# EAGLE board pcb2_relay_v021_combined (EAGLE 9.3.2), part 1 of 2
2022-05-20: PCB made by JLCPCB
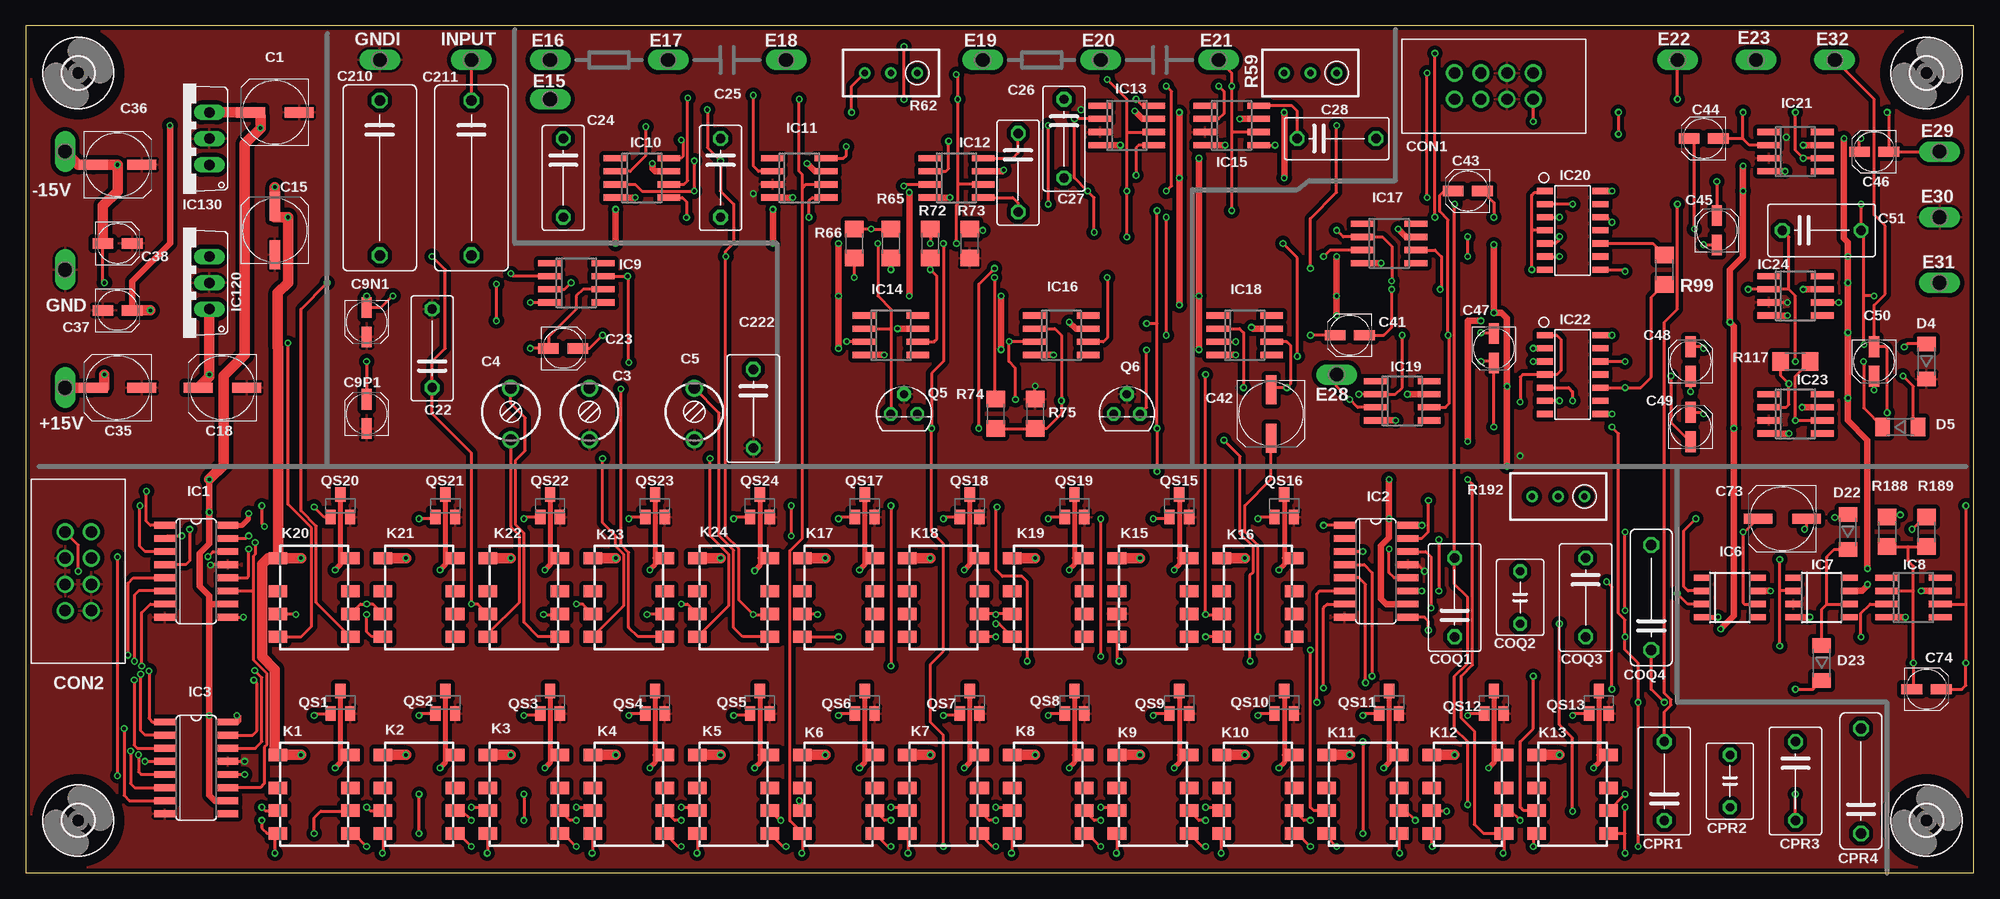
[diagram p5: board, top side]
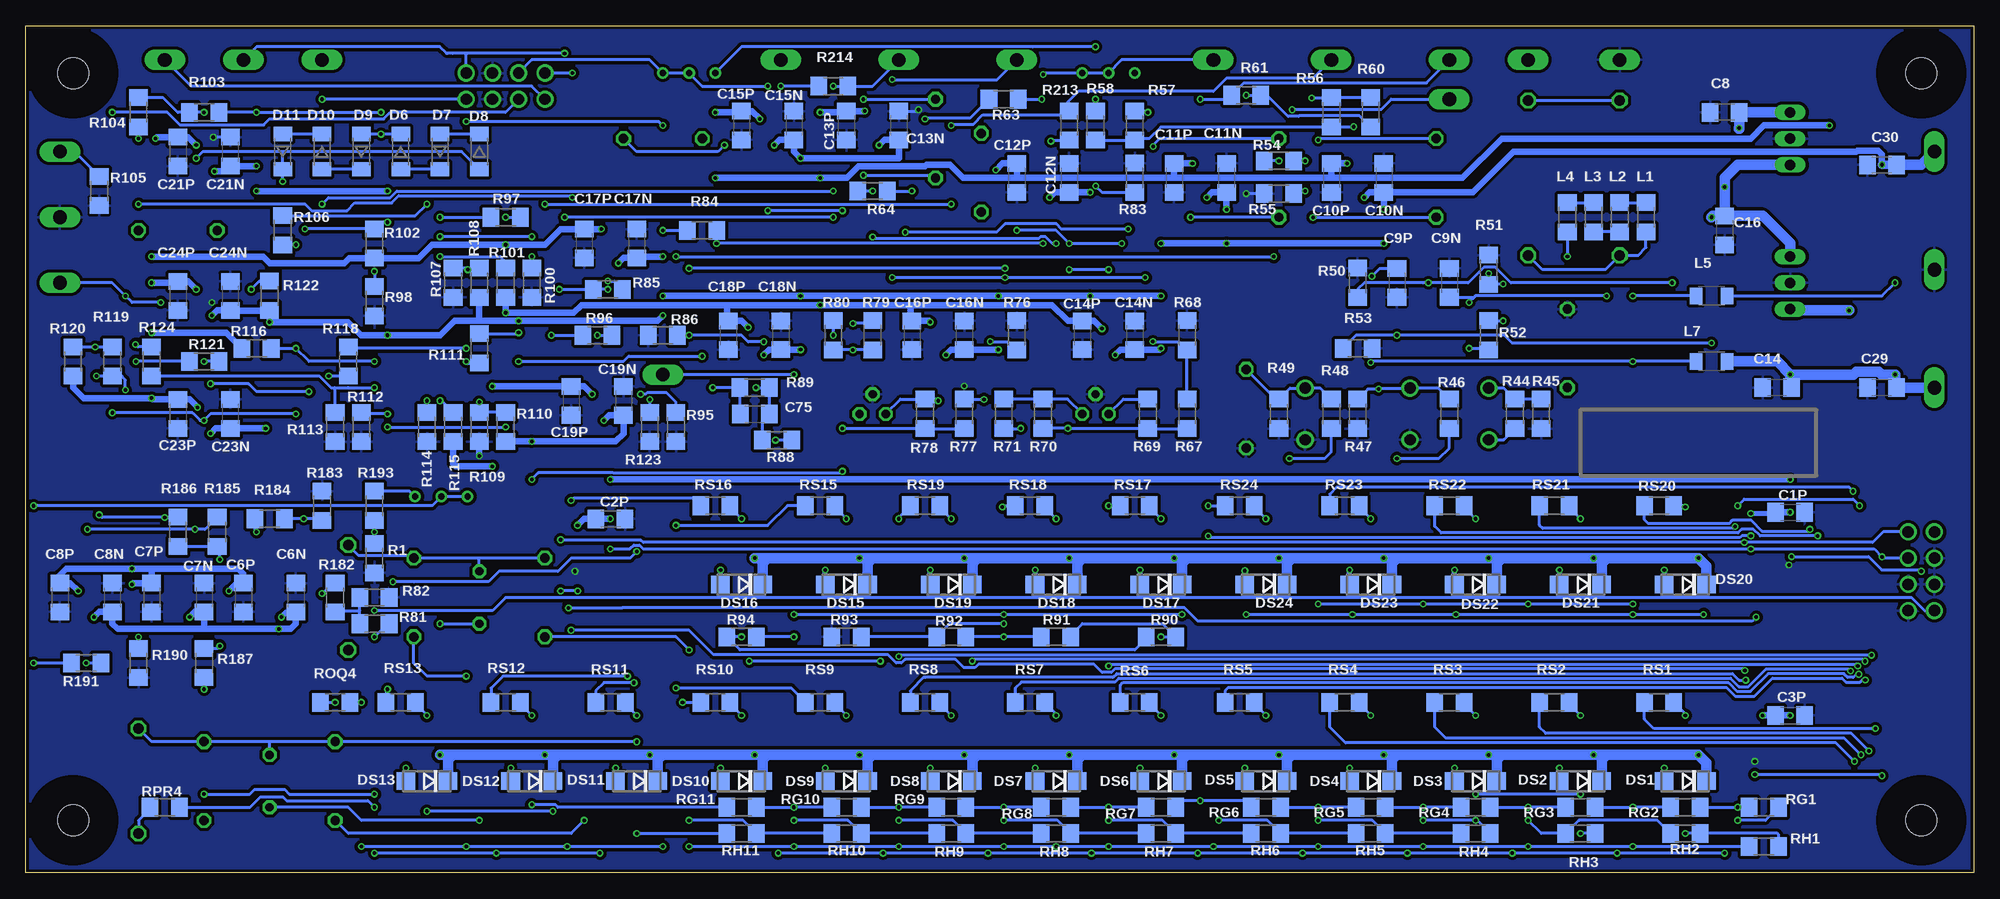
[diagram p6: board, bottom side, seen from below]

Size 188.72 x 82.04 mm. Coordinates in mm from the lower left corner, seen from the top.
Outline: 0,0 188.72,0 188.72,82.04 0,82.04 0,0
Copper layers (1*16): Top 0.035mm / dielectric 1.5mm / Bottom 0.035mm
Design rules "ITEADstudio_DRC for Eagle v6": minimum track width 6mil, minimum drill 12mil, track to track 6mil, track to pad 6mil, pad to pad 6mil, via to via 6mil, smd to smd 0mil, copper to edge 10mil, drill to drill 10mil, minimum pad ring 10mil, minimum via ring 6mil, stop-mask expansion 2mil, vias tented up to drill 100mil, thermal gap 10mil

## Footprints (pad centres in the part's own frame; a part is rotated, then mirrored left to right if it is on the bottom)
P1-13Y = drill 1.321 pad 1.905 long: TP 0,0
UD-6,3X5,8_NICHICON = smd 2.8 x 1: + 2.35,0; - -2.35,0
C1206 = smd 1.6 x 1.8: 1 -1.4,0; 2 1.4,0
CTRIM3050.504 = drill 1.1: 1 -2.5,0; 2 2.5,0
UD-4X5,8_NICHICON = smd 2 x 1: + 1.425,0; - -1.425,0
C075-042X103 = drill 0.914 octagon: 1 -3.81,0; 2 3.81,0
C075-052X106 = drill 0.914 octagon: 1 -3.81,0; 2 3.81,0
C150-072X183 = drill 1.016 octagon: 1 -7.493,0; 2 7.493,0
61200821621 = drill 1.1: 1 -2.54,-1.27; 2 -2.54,1.27; 3 0,-1.27; 4 0,1.27; 5 2.54,-1.27; 6 2.54,1.27; 7 5.08,-1.27; 8 5.08,1.27
C050-045X075 = drill 0.813 octagon: 1 -2.54,0; 2 2.54,0
C102-043X133 = drill 1.016 octagon: 1 -5.08,0; 2 5.08,0
SOD80 = smd 1.4 x 1.8: 1 -1.7,0; 2 1.7,0
DO214AC = smd 1.8 x 1.7: A 2.05,0; C -2.05,0
SO16 = smd 0.66 x 2.032: 1 -4.445,-3.073; 2 -3.175,-3.073; 3 -1.905,-3.073; 4 -0.635,-3.073; 5 0.635,-3.073; 6 1.905,-3.073; 7 3.175,-3.073; 8 4.445,-3.073; 9 4.445,3.073; 10 3.175,3.073; 11 1.905,3.073; 12 0.635,3.073; 13 -0.635,3.073; 14 -1.905,3.073; 15 -3.175,3.073; 16 -4.445,3.073
SOIC8 = smd 0.6 x 1.5: 1 -1.905,-2.75; 2 -0.635,-2.75; 3 0.635,-2.75; 4 1.905,-2.75; 5 1.905,2.75; 6 0.635,2.75; 7 -0.635,2.75; 8 -1.905,2.75
SO08 = smd 0.6 x 2.2: 1 -1.905,-2.6; 2 -0.635,-2.6; 3 0.635,-2.6; 4 1.905,-2.6; 5 1.905,2.6; 6 0.635,2.6; 7 -0.635,2.6; 8 -1.905,2.6
SOIC-14 = smd 0.6 x 1.55: 1 -3.81,-2.7; 2 -2.54,-2.7; 3 -1.27,-2.7; 4 0,-2.7; 5 1.27,-2.7; 6 2.54,-2.7; 7 3.81,-2.7; 8 3.81,2.7; 9 2.54,2.7; 10 1.27,2.7; 11 0,2.7; 12 -1.27,2.7; 13 -2.54,2.7; 14 -3.81,2.7
TO220V = drill 1.016 long: 1 -2.54,-2.54; 2 0,-2.54; 3 2.54,-2.54
G6K-2F-Y = smd 1.2 x 1.8: 1 -3.8,-3.5; 2 -0.6,-3.5; 3 1.6,-3.5; 4 3.8,-3.5; 5 3.8,3.5; 6 1.6,3.5; 7 -0.6,3.5; 8 -3.8,3.5
FB1206 = smd 1.6 x 1.803: 1 -1.422,0; 2 1.422,0
L3216C = smd 1.2 x 1.6: 1 -1.5,0; 2 1.5,0
TO92G = drill 0.813 octagon: D -1.27,0; G 1.27,0; S 0,1.905
SOT23 = smd 1 x 1.4: 1 -0.95,-1.1; 2 0.95,-1.1; 3 0,1.1
R1206 = smd 1.6 x 1.803: 1 -1.422,0; 2 1.422,0
RTRIM3296W = drill 0.61: 1 0,-2.54; 2 0,0; 3 0,2.54
3,0 = hole 3: 0,0

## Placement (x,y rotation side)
+15V  TPPAD1-13Y  [P1-13Y]  3.81,46.99 0 top
-15V  TPPAD1-13Y  [P1-13Y]  3.81,69.85 0 top
C1  100u/16V  [UD-6,3X5,8_NICHICON]  24.13,73.66 180 top
C1P  100n  [C1206]  17.78,34.92 0 bottom
C2P  100n  [C1206]  132.08,34.29 0 bottom
C3  30p  [CTRIM3050.504]  54.61,44.45 90 top
C3P  100n  [C1206]  17.78,15.24 0 bottom
C4  5p  [CTRIM3050.504]  46.99,44.45 90 top
C5  30p  [CTRIM3050.504]  64.77,44.45 90 top
C6N  100n  [C1206]  162.56,26.67 270 bottom
C6P  100n  [C1206]  167.64,26.67 270 bottom
C7N  100n  [C1206]  171.45,26.67 270 bottom
C7P  100n  [C1206]  176.53,26.67 270 bottom
C8  100n  [C1206]  24.13,73.66 180 bottom
C8N  100n  [C1206]  180.34,26.67 270 bottom
C8P  100n  [C1206]  185.42,26.67 270 bottom
C9N  100n  [C1206]  50.8,57.15 270 bottom
C9N1  10u/25V  [UD-4X5,8_NICHICON]  33.02,53.34 270 top
C9P  100n  [C1206]  55.88,57.15 270 bottom
C9P1  10u/25V  [UD-4X5,8_NICHICON]  33.02,44.45 90 top
C10N  100n  [C1206]  57.15,67.31 270 bottom
C10P  100n  [C1206]  62.23,67.31 270 bottom
C11N  100n  [C1206]  72.39,67.31 270 bottom
C11P  100n  [C1206]  77.47,67.31 270 bottom
C12N  100n  [C1206]  87.63,67.31 270 bottom
C12P  100n  [C1206]  92.71,67.31 270 bottom
C13N  100n  [C1206]  104.14,72.39 270 bottom
C13P  100n  [C1206]  109.22,72.39 270 bottom
C14  100n  [C1206]  19.05,46.99 180 bottom
C14N  100n  [C1206]  81.28,52.07 270 bottom
C14P  100n  [C1206]  86.36,52.07 270 bottom
C15  100u/16V  [UD-6,3X5,8_NICHICON]  24.13,62.23 90 top
C15N  100n  [C1206]  114.3,72.39 270 bottom
C15P  100n  [C1206]  119.38,72.39 270 bottom
C16  100n  [C1206]  24.13,62.23 270 bottom
C16N  100n  [C1206]  97.79,52.07 270 bottom
C16P  100n  [C1206]  102.87,52.07 270 bottom
C17N  100n  [C1206]  129.54,60.96 270 bottom
C17P  100n  [C1206]  134.62,60.96 270 bottom
C18  100u/16V  [UD-6,3X5,8_NICHICON]  19.05,46.99 180 top
C18N  100n  [C1206]  115.57,52.07 270 bottom
C18P  100n  [C1206]  120.65,52.07 270 bottom
C19N  100n  [C1206]  130.81,45.72 270 bottom
C19P  100n  [C1206]  135.89,45.72 270 bottom
C21N  100n  [C1206]  168.91,69.85 270 bottom
C21P  100n  [C1206]  173.99,69.85 270 bottom
C22  47p  [C075-042X103]  39.37,50.8 90 top
C23  10u/25V  [UD-4X5,8_NICHICON]  52.07,50.8 0 top
C23N  100n  [C1206]  168.91,44.45 270 bottom
C23P  100n  [C1206]  173.99,44.45 270 bottom
C24  10p  [C075-042X103]  52.07,67.31 270 top
C24N  100n  [C1206]  168.91,55.88 270 bottom
C24P  100n  [C1206]  173.99,55.88 270 bottom
C25  15p  [C075-042X103]  67.31,67.31 270 top
C26  22p  [C075-042X103]  96.14,67.82 270 top
C27  15p  [C075-042X103]  100.58,71.12 270 top
C28  22p  [C075-042X103]  127,71.12 0 top
C29  100n  [C1206]  8.89,46.99 180 bottom
C30  100n  [C1206]  8.89,68.58 0 bottom
C35  100u/16V  [UD-6,3X5,8_NICHICON]  8.89,46.99 180 top
C36  100u/16V  [UD-6,3X5,8_NICHICON]  8.89,68.58 0 top
C37  1u/50V  [UD-4X5,8_NICHICON]  8.89,54.48 0 top
C38  1u/50V  [UD-4X5,8_NICHICON]  8.89,60.96 0 top
C41  10u/25V  [UD-4X5,8_NICHICON]  128.27,52.07 180 top
C42  100u/16V  [UD-6,3X5,8_NICHICON]  120.65,44.45 270 top
C43  10u/25V  [UD-4X5,8_NICHICON]  139.7,66.04 180 top
C44  1u/50V  [UD-4X5,8_NICHICON]  162.56,71.12 180 top
C45  10u/25V  [UD-4X5,8_NICHICON]  163.83,62.23 90 top
C46  10u/25V  [UD-4X5,8_NICHICON]  179.07,69.85 180 top
C47  10u/25V  [UD-4X5,8_NICHICON]  142.24,50.8 270 top
C48  1u/50V  [UD-4X5,8_NICHICON]  161.29,49.53 90 top
C49  10u/25V  [UD-4X5,8_NICHICON]  161.29,43.18 90 top
C50  1u/50V  [UD-4X5,8_NICHICON]  179.07,49.53 270 top
C51  220n  [C075-052X106]  173.99,62.23 0 top
C73  100u/16V  [UD-6,3X5,8_NICHICON]  170.18,34.29 180 top
C74  1u/50V  [UD-4X5,8_NICHICON]  184.15,17.78 0 top
C75  2p  [C1206]  118.11,44.45 0 bottom
C210  1u  [C150-072X183]  34.29,67.31 270 top
C211  1u  [C150-072X183]  43.18,67.31 270 top
C222  68p  [C075-052X106]  70.48,44.96 270 top
CON1  PCB2_IO  [61200821621]  140.97,76.2 0 top
CON2  UC_IO  [61200821621]  5.08,27.94 90 top
COQ1  220n  [C075-052X106]  138.43,26.67 90 top
COQ2  22n  [C050-045X075]  144.78,26.67 90 top
COQ3  2n2  [C075-052X106]  151.13,26.67 270 top
COQ4  200p  [C102-043X133]  157.48,26.67 90 top
CPR1  220n  [C075-052X106]  158.75,8.89 90 top
CPR2  22n  [C050-045X075]  165.1,8.89 90 top
CPR3  2n2  [C075-052X106]  171.45,8.89 270 top
CPR4  200p  [C102-043X133]  177.8,8.89 90 top
D4  1N4148  [SOD80]  184.15,49.53 90 top
D5  1N4148  [SOD80]  181.61,43.18 0 top
D6  1N4148  [SOD80]  152.4,69.85 270 bottom
D7  1N4148  [SOD80]  148.59,69.85 90 bottom
D8  1N4148  [SOD80]  144.78,69.85 270 bottom
D9  1N4148  [SOD80]  156.21,69.85 90 bottom
D10  1N4148  [SOD80]  160.02,69.85 270 bottom
D11  1N4148  [SOD80]  163.83,69.85 90 bottom
D22  1N4148  [SOD80]  176.53,33.02 90 top
D23  1N4148  [SOD80]  173.99,20.32 90 top
DS1  M7  [DO214AC]  27.94,8.89 180 bottom
DS2  M7  [DO214AC]  38.1,8.89 180 bottom
DS3  M7  [DO214AC]  48.26,8.89 180 bottom
DS4  M7  [DO214AC]  58.42,8.89 180 bottom
DS5  M7  [DO214AC]  68.58,8.89 180 bottom
DS6  M7  [DO214AC]  78.74,8.89 180 bottom
DS7  M7  [DO214AC]  88.9,8.89 180 bottom
DS8  M7  [DO214AC]  99.06,8.89 180 bottom
DS9  M7  [DO214AC]  109.22,8.89 180 bottom
DS10  M7  [DO214AC]  119.38,8.89 180 bottom
DS11  M7  [DO214AC]  129.54,8.89 180 bottom
DS12  M7  [DO214AC]  139.7,8.89 180 bottom
DS13  M7  [DO214AC]  149.86,8.89 180 bottom
DS15  M7  [DO214AC]  109.22,27.94 180 bottom
DS16  M7  [DO214AC]  119.38,27.94 180 bottom
DS17  M7  [DO214AC]  78.74,27.94 180 bottom
DS18  M7  [DO214AC]  88.9,27.94 180 bottom
DS19  M7  [DO214AC]  99.06,27.94 180 bottom
DS20  M7  [DO214AC]  27.94,27.94 180 bottom
DS21  M7  [DO214AC]  38.1,27.94 180 bottom
DS22  M7  [DO214AC]  48.26,27.94 180 bottom
DS23  M7  [DO214AC]  58.42,27.94 180 bottom
DS24  M7  [DO214AC]  68.58,27.94 180 bottom
E15  TPPAD1-13Y  [P1-13Y]  50.8,74.93 90 top
E16  TPPAD1-13Y  [P1-13Y]  50.8,78.74 90 top
E17  TPPAD1-13Y  [P1-13Y]  62.23,78.74 90 top
E18  TPPAD1-13Y  [P1-13Y]  73.66,78.74 90 top
E19  TPPAD1-13Y  [P1-13Y]  92.71,78.74 90 top
E20  TPPAD1-13Y  [P1-13Y]  104.14,78.74 270 top
E21  TPPAD1-13Y  [P1-13Y]  115.57,78.74 270 top
E22  TPPAD1-13Y  [P1-13Y]  160.02,78.74 90 top
E23  TPPAD1-13Y  [P1-13Y]  167.64,78.74 90 top
E28  TPPAD1-13Y  [P1-13Y]  127,48.26 270 top
E29  TPPAD1-13Y  [P1-13Y]  185.42,69.85 90 top
E30  TPPAD1-13Y  [P1-13Y]  185.42,63.5 90 top
E31  TPPAD1-13Y  [P1-13Y]  185.42,57.15 90 top
E32  TPPAD1-13Y  [P1-13Y]  175.26,78.74 90 top
GND  TPPAD1-13Y  [P1-13Y]  3.81,58.42 0 top
GNDI  TPPAD1-13Y  [P1-13Y]  34.29,78.74 90 top
IC1  74HC595D  [SO16]  16.51,29.21 270 top
IC2  74HC595D  [SO16]  130.81,29.21 270 top
IC3  74HC595D  [SO16]  16.51,10.16 270 top
IC6  LM318D  [SOIC8]  165.1,26.67 270 top
IC7  LM318D  [SOIC8]  173.99,26.67 270 top
IC8  LM741D  [SO08]  182.88,26.67 270 top
IC9  NE5534AD  [SO08]  53.34,57.15 270 top
IC10  NE5534AD  [SO08]  59.69,67.31 270 top
IC11  NE5534AD  [SO08]  74.93,67.31 270 top
IC12  NE5534AD  [SO08]  90.17,67.31 270 top
IC13  NE5534AD  [SO08]  106.68,72.39 270 top
IC14  NE5534AD  [SO08]  83.82,52.07 270 top
IC15  NE5534AD  [SO08]  116.84,72.39 270 top
IC16  NE5534AD  [SO08]  100.33,52.07 270 top
IC17  NE5534AD  [SO08]  132.08,60.96 270 top
IC18  LM318D  [SO08]  118.11,52.07 270 top
IC19  LM318D  [SO08]  133.35,45.72 270 top
IC20  MC1496D  [SOIC-14]  149.86,62.23 270 top
IC21  LM318D  [SO08]  171.45,69.85 270 top
IC22  MC1496D  [SOIC-14]  149.86,48.26 270 top
IC23  LM318D  [SO08]  171.45,44.45 270 top
IC24  LF356D  [SO08]  171.45,55.88 270 top
IC120  7812TV  [TO220V]  15.24,57.15 90 top
IC130  7805TV  [TO220V]  15.24,71.12 90 top
INPUT  TPPAD1-13Y  [P1-13Y]  43.18,78.74 90 top
K1  G6K-2F-Y  [G6K-2F-Y]  27.94,7.62 270 top
K2  G6K-2F-Y  [G6K-2F-Y]  38.1,7.62 270 top
K3  G6K-2F-Y  [G6K-2F-Y]  48.26,7.62 270 top
K4  G6K-2F-Y  [G6K-2F-Y]  58.42,7.62 270 top
K5  G6K-2F-Y  [G6K-2F-Y]  68.58,7.62 270 top
K6  G6K-2F-Y  [G6K-2F-Y]  78.74,7.62 270 top
K7  G6K-2F-Y  [G6K-2F-Y]  88.9,7.62 270 top
K8  G6K-2F-Y  [G6K-2F-Y]  99.06,7.62 270 top
K9  G6K-2F-Y  [G6K-2F-Y]  109.22,7.62 270 top
K10  G6K-2F-Y  [G6K-2F-Y]  119.38,7.62 270 top
K11  G6K-2F-Y  [G6K-2F-Y]  129.54,7.62 270 top
K12  G6K-2F-Y  [G6K-2F-Y]  139.7,7.62 270 top
K13  G6K-2F-Y  [G6K-2F-Y]  149.86,7.62 270 top
K15  G6K-2F-Y  [G6K-2F-Y]  109.22,26.67 270 top
K16  G6K-2F-Y  [G6K-2F-Y]  119.38,26.67 270 top
K17  G6K-2F-Y  [G6K-2F-Y]  78.74,26.67 270 top
K18  G6K-2F-Y  [G6K-2F-Y]  88.9,26.67 270 top
K19  G6K-2F-Y  [G6K-2F-Y]  99.06,26.67 270 top
K20  G6K-2F-Y  [G6K-2F-Y]  27.94,26.67 270 top
K21  G6K-2F-Y  [G6K-2F-Y]  38.1,26.67 270 top
K22  G6K-2F-Y  [G6K-2F-Y]  48.26,26.67 270 top
K23  G6K-2F-Y  [G6K-2F-Y]  58.42,26.67 270 top
K24  G6K-2F-Y  [G6K-2F-Y]  68.58,26.67 270 top
L1  600  [FB1206]  31.75,63.5 270 bottom
L2  600  [FB1206]  34.29,63.5 270 bottom
L3  600  [FB1206]  36.83,63.5 270 bottom
L4  600  [FB1206]  39.37,63.5 270 bottom
L5  10u  [L3216C]  25.4,55.88 180 bottom
L7  10u  [L3216C]  25.4,49.53 180 bottom
Q5  2N4091  [TO92G]  85.09,44.45 0 top
Q6  2N4091  [TO92G]  106.68,44.45 0 top
QS1  SS8050  [SOT23]  30.48,16.51 0 top
QS2  SS8050  [SOT23]  40.64,16.51 0 top
QS3  SS8050  [SOT23]  50.8,16.51 0 top
QS4  SS8050  [SOT23]  60.96,16.51 0 top
QS5  SS8050  [SOT23]  71.12,16.51 0 top
QS6  SS8050  [SOT23]  81.28,16.51 0 top
QS7  SS8050  [SOT23]  91.44,16.51 0 top
QS8  SS8050  [SOT23]  101.6,16.51 0 top
QS9  SS8050  [SOT23]  111.76,16.51 0 top
QS10  SS8050  [SOT23]  121.92,16.51 0 top
QS11  SS8050  [SOT23]  132.08,16.51 0 top
QS12  SS8050  [SOT23]  142.24,16.51 0 top
QS13  SS8050  [SOT23]  152.4,16.51 0 top
QS15  SS8050  [SOT23]  111.76,35.56 0 top
QS16  SS8050  [SOT23]  121.92,35.56 0 top
QS17  SS8050  [SOT23]  81.28,35.56 0 top
QS18  SS8050  [SOT23]  91.44,35.56 0 top
QS19  SS8050  [SOT23]  101.6,35.56 0 top
QS20  SS8050  [SOT23]  30.48,35.56 0 top
QS21  SS8050  [SOT23]  40.64,35.56 0 top
QS22  SS8050  [SOT23]  50.8,35.56 0 top
QS23  SS8050  [SOT23]  60.96,35.56 0 top
QS24  SS8050  [SOT23]  71.12,35.56 0 top
R1  3K3  [R1206]  154.94,30.48 90 bottom
R44  68K1  [R1206]  44.45,44.45 90 bottom
R45  42K2  [R1206]  41.91,44.45 90 bottom
R46  90K9  [R1206]  50.8,44.45 90 bottom
R47  11K  [R1206]  59.69,44.45 90 bottom
R48  100K  [R1206]  62.23,44.45 90 bottom
R49  3K16  [R1206]  67.31,44.45 90 bottom
R50  100K  [R1206]  59.69,57.15 270 bottom
R51  1K  [R1206]  46.99,58.42 270 bottom
R52  2K05  [R1206]  46.99,52.07 270 bottom
R53  1M  [R1206]  59.69,50.8 180 bottom
R54  82K  [R1206]  67.31,68.96 180 bottom
R55  18K  [R1206]  67.31,65.79 0 bottom
R56  10K  [R1206]  62.23,73.66 90 bottom
R57  22k  [R1206]  81.28,72.39 90 bottom
R58  6K8  [R1206]  85.09,72.39 90 bottom
R59  5K  [RTRIM3296W]  124.46,77.47 90 top
R60  10K  [R1206]  58.42,73.66 270 bottom
R61  10K  [R1206]  70.48,75.31 180 bottom
R62  5K  [RTRIM3296W]  83.82,77.47 90 top
R63  10K  [R1206]  93.98,74.93 0 bottom
R64  10K  [R1206]  106.68,66.04 180 bottom
R65  82K  [R1206]  83.82,60.96 270 top
R66  150K  [R1206]  80.26,60.96 90 top
R67  10K  [R1206]  76.2,44.45 270 bottom
R68  270  [R1206]  76.2,52.07 270 bottom
R69  1K5  [R1206]  80.01,44.45 270 bottom
R70  750K  [R1206]  90.17,44.45 270 bottom
R71  10K  [R1206]  93.98,44.45 90 bottom
R72  560  [R1206]  87.63,60.96 270 top
R73  330  [R1206]  91.44,60.96 90 top
R74  560  [R1206]  93.98,44.45 90 top
R75  330  [R1206]  97.79,44.45 270 top
R76  270  [R1206]  92.71,52.07 270 bottom
R77  10K  [R1206]  97.79,44.45 270 bottom
R78  1K5  [R1206]  101.6,44.45 270 bottom
R79  750K  [R1206]  106.68,52.07 90 bottom
R80  10K  [R1206]  110.49,52.07 270 bottom
R81  27K  [R1206]  154.94,24.13 180 bottom
R82  4K7  [R1206]  154.94,26.67 0 bottom
R83  100  [R1206]  81.28,67.31 270 bottom
R84  2K2  [R1206]  123.19,62.23 0 bottom
R85  18K  [R1206]  132.33,56.52 0 bottom
R86  100K  [R1206]  127,52.07 0 bottom
R88  1K1  [R1206]  115.95,41.91 0 bottom
R89  10K  [R1206]  118.11,46.99 0 bottom
R90  7K5  [R1206]  78.74,22.86 0 bottom
R91  2K15  [R1206]  88.9,22.86 180 bottom
R92  750  [R1206]  99.06,22.86 180 bottom
R93  316  [R1206]  109.22,22.86 180 bottom
R94  6K2  [R1206]  119.38,22.86 180 bottom
R95  1K1  [R1206]  125.73,43.18 270 bottom
R96  10K  [R1206]  133.35,52.07 0 bottom
R97  15K  [R1206]  142.24,63.5 0 bottom
R98  100  [R1206]  154.94,55.37 270 bottom
R99  100  [R1206]  158.75,58.42 270 top
R100  15K  [R1206]  139.7,57.15 270 bottom
R101  100  [R1206]  142.24,57.15 90 bottom
R102  6K8  [R1206]  154.94,60.96 270 bottom
R103  1M  [R1206]  171.45,73.66 180 bottom
R104  470  [R1206]  177.8,73.66 270 bottom
R105  100K  [R1206]  181.61,66.04 270 bottom
R106  15K  [R1206]  163.83,62.23 270 bottom
R107  4K7  [R1206]  147.32,57.15 90 bottom
R108  4K7  [R1206]  144.78,57.15 270 bottom
R109  4K7  [R1206]  144.78,43.18 90 bottom
R110  4K7  [R1206]  142.24,43.18 270 bottom
R111  15K  [R1206]  144.78,50.8 90 bottom
R112  100  [R1206]  156.21,43.18 270 bottom
R113  100  [R1206]  158.75,43.18 270 bottom
R114  15K  [R1206]  149.86,43.18 270 bottom
R115  100  [R1206]  147.32,43.18 90 bottom
R116  6K8  [R1206]  166.37,50.8 180 bottom
R117  1M  [R1206]  171.45,49.53 0 top
R118  15K  [R1206]  157.48,49.53 270 bottom
R119  100K  [R1206]  180.34,49.53 270 bottom
R120  100K  [R1206]  184.15,49.53 90 bottom
R121  1M  [R1206]  171.45,49.53 0 bottom
R122  22M  [R1206]  165.1,55.88 90 bottom
R123  100K  [R1206]  128.27,43.18 90 bottom
R124  11K  [R1206]  176.53,49.53 90 bottom
R182  100  [R1206]  158.75,26.67 270 bottom
R183  1K  [R1206]  160.02,35.56 90 bottom
R184  1K  [R1206]  165.1,34.29 0 bottom
R185  1K  [R1206]  170.18,33.02 90 bottom
R186  1K  [R1206]  173.99,33.02 90 bottom
R187  1K  [R1206]  171.45,20.32 90 bottom
R188  10K  [R1206]  180.34,33.02 270 top
R189  20K  [R1206]  184.15,33.02 90 top
R190  6K8  [R1206]  177.8,20.32 90 bottom
R191  270K  [R1206]  182.88,20.32 180 bottom
R192  5K  [RTRIM3296W]  148.46,36.45 90 top
R193  4K7  [R1206]  154.94,35.56 90 bottom
R213  220  [R1206]  87.63,72.39 270 bottom
R214  220  [R1206]  110.49,76.2 180 bottom
RG1  7K5  [R1206]  20.32,6.35 180 bottom
RG2  5K62  [R1206]  27.94,6.35 180 bottom
RG3  6K19  [R1206]  38.1,6.35 180 bottom
RG4  3K83  [R1206]  48.26,6.35 180 bottom
RG5  3K48  [R1206]  58.42,6.35 180 bottom
RG6  2K15  [R1206]  68.58,6.35 180 bottom
RG7  1K96  [R1206]  78.74,6.35 180 bottom
RG8  1K78  [R1206]  88.9,6.35 180 bottom
RG9  1K1  [R1206]  99.06,6.35 180 bottom
RG10  1K  [R1206]  109.22,6.35 180 bottom
RG11  3K83  [R1206]  119.38,6.35 180 bottom
RH1  7K5  [R1206]  20.32,2.54 0 bottom
RH2  5K62  [R1206]  27.94,3.81 180 bottom
RH3  6K19  [R1206]  38.1,3.81 0 bottom
RH4  3K83  [R1206]  48.26,3.81 180 bottom
RH5  3K48  [R1206]  58.42,3.81 180 bottom
RH6  2K15  [R1206]  68.58,3.81 180 bottom
RH7  1K96  [R1206]  78.74,3.81 180 bottom
RH8  1K78  [R1206]  88.9,3.81 180 bottom
RH9  1K1  [R1206]  99.06,3.81 180 bottom
RH10  1K  [R1206]  109.22,3.81 180 bottom
RH11  3K83  [R1206]  119.38,3.81 180 bottom
ROQ4  180  [R1206]  158.75,16.51 180 bottom
RPR4  180  [R1206]  175.26,6.35 180 bottom
RS1  4K7  [R1206]  30.48,16.51 180 bottom
RS2  4K7  [R1206]  40.64,16.51 180 bottom
RS3  4K7  [R1206]  50.8,16.51 180 bottom
RS4  4K7  [R1206]  60.96,16.51 180 bottom
RS5  4K7  [R1206]  71.12,16.51 180 bottom
RS6  4K7  [R1206]  81.28,16.51 180 bottom
RS7  4K7  [R1206]  91.44,16.51 180 bottom
RS8  4K7  [R1206]  101.6,16.51 180 bottom
RS9  4K7  [R1206]  111.76,16.51 180 bottom
RS10  4K7  [R1206]  121.92,16.51 180 bottom
RS11  4K7  [R1206]  132.08,16.51 180 bottom
RS12  4K7  [R1206]  142.24,16.51 180 bottom
RS13  4K7  [R1206]  152.4,16.51 180 bottom
RS15  4K7  [R1206]  111.76,35.56 180 bottom
RS16  4K7  [R1206]  121.92,35.56 180 bottom
RS17  4K7  [R1206]  81.28,35.56 180 bottom
RS18  4K7  [R1206]  91.44,35.56 180 bottom
RS19  4K7  [R1206]  101.6,35.56 180 bottom
RS20  4K7  [R1206]  30.48,35.56 180 bottom
RS21  4K7  [R1206]  40.64,35.56 180 bottom
RS22  4K7  [R1206]  50.8,35.56 180 bottom
RS23  4K7  [R1206]  60.96,35.56 180 bottom
RS24  4K7  [R1206]  71.12,35.56 180 bottom
U$1  [3,0]  5.08,5.08 0 top
U$2  [3,0]  5.08,77.47 0 top
U$3  [3,0]  184.15,77.47 0 top
U$4  [3,0]  184.15,5.08 0 top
